|Texas Instruments Incorporated
|IWRL6432 Single-Chip 60GHz mmWave Sensor
[IBIS Ver]   5.0
[Comment Char] |_char
[File name]   iwrl6432_wcsp111.ibs
[Date]   12/10/2024
[File Rev]   1.0
[Source]   Cadence Layout Workbench 22.1.4.12161.401368   004
[Notes]   Revision History:
| Rev 1.0: 12/10/2024
| - Initial version of the model
[Disclaimer]
| This model is designed as an aid for customers of Texas Instruments.
| TI and its licensors and suppliers make no warranties, either expressed
| or implied, with respect to this  model, including the warranties of
| merchantability or fitness for a particular purpose. The model is
| provided solely on an "as is" basis. The entire risk as to its quality
| and performance is with the customer.
| This model is subject to change without notice. Texas Instruments
| Incorporated is not responsible for updating this model.
[Copyright]
(C) Copyright 2024 Texas Instruments Incorporated.All rights reserved.
|  Component IWRL6432BDQGYFFR 111-pin - YFF0111 package
|  Part # IWRL6432BDQGYFFR
[Component]   IWRL6432BDQGYFFR
[Manufacturer]   Texas Instruments
[Package]   |111 WCSP - YFF0111 package
|  variable   typ   min   max
R_pkg   0.12533   0.026709   0.27962
L_pkg   3.002e-10   1.085e-10   5.3e-10
C_pkg   3.033e-13   2.488e-13   4.027e-13
[Pin]   signal_name   model_name   R_pin   L_pin   C_pin
A1   VSSA   GND   NA   NA   NA
A2   TX1   NC   NA   NA   NA
A3   VSSA   GND   NA   NA   NA
A4   TX2   NC   NA   NA   NA
A5   VSSA   GND   NA   NA   NA
A6   VIOIN_18   POWER   NA   NA   NA
A7   VSS   GND   NA   NA   NA
A8   VDD   POWER   NA   NA   NA
A9   QSPI[2]   IO2   NA   NA   NA
A10   QSPI[3]   IO2   NA   NA   NA
A11   VSS   GND   NA   NA   NA
B1   VSSA   GND   NA   NA   NA
B2   VSSA   GND   NA   NA   NA
B4   VSSA   GND   NA   NA   NA
B5   VSSA   GND   NA   NA   NA
B6   VPP   POWER   NA   NA   NA
B7   VSS   GND   NA   NA   NA
B8   VDD   POWER   NA   NA   NA
B9   QSPI_CS   IO2   NA   NA   NA
B10   QSPI[0]   IO2   NA   NA   NA
B11   QSPI[1]   IO2   NA   NA   NA
C1   CLKM   NC   NA   NA   NA
C5   VSSA_PM   NC   NA   NA   NA
C6   VDD   POWER   NA   NA   NA
C7   VDD   POWER   NA   NA   NA
C8   VDD   POWER   NA   NA   NA
C9   SPIA_MOSI   IO2   NA   NA   NA
C10   SPIA_MISO   IO2   NA   NA   NA
C11   QSPI_CLK   IO2   NA   NA   NA
D1   CLKP   NC   NA   NA   NA
D2   VOUT_14SYNTH   NC   NA   NA   NA
D3   VDDA_10RF   POWER   NA   NA   NA
D4   VDDA_10RF   POWER   NA   NA   NA
D5   OSC_CLK_OUT   NC   NA   NA   NA
D6   VDD   POWER   NA   NA   NA
D7   VDD   POWER   NA   NA   NA
D8   VDD   POWER   NA   NA   NA
D9   VDD   POWER   NA   NA   NA
D10   SPIA_CS0_N   IO2   NA   NA   NA
D11   SPIA_CLK   IO2   NA   NA   NA
E1   VSSA   GND   NA   NA   NA
E2   VSSA   GND   NA   NA   NA
E6   VDD   POWER   NA   NA   NA
E7   VDD   POWER   NA   NA   NA
E8   VDD   POWER   NA   NA   NA
E9   VDD   POWER   NA   NA   NA
E10   TCK   IO2   NA   NA   NA
E11   VIOIN   POWER   NA   NA   NA
F1   RX3   NC   NA   NA   NA
F2   VSSA   GND   NA   NA   NA
F3   VDDA_18VCO   POWER   NA   NA   NA
F4   VIN_18PM   POWER   NA   NA   NA
F5   VIOIN_18CLK   POWER   NA   NA   NA
F6   VSS   GND   NA   NA   NA
F7   VSS   GND   NA   NA   NA
F8   VSS   GND   NA   NA   NA
F9   VSS   GND   NA   NA   NA
F10   TDI   IO2   NA   NA   NA
F11   TDO   IO2   NA   NA   NA
G1   VSSA   GND   NA   NA   NA
G2   VSSA   GND   NA   NA   NA
G3   VOUT_14APLL   NC   NA   NA   NA
G4   VDDA_18BB   POWER   NA   NA   NA
G5   VSS   GND   NA   NA   NA
G6   VSS   GND   NA   NA   NA
G7   VSS   GND   NA   NA   NA
G8   VSS   GND   NA   NA   NA
G9   VSS   GND   NA   NA   NA
G10   TMS   IO2   NA   NA   NA
G11   VIOIN_18   POWER   NA   NA   NA
H1   RX2   NC   NA   NA   NA
H2   VSSA   GND   NA   NA   NA
H3   VDDA_10RF   POWER   NA   NA   NA
H4   VBGAP   NC   NA   NA   NA
H6   VSS   GND   NA   NA   NA
H7   VSS   GND   NA   NA   NA
H8   VSS   GND   NA   NA   NA
H9   VSS   GND   NA   NA   NA
H10   RS232_TX   IO2   NA   NA   NA
H11   RS232_RX   IO2   NA   NA   NA
J1   VSSA   GND   NA   NA   NA
J2   VSSA   GND   NA   NA   NA
J3   VDDA_10RF   POWER   NA   NA   NA
J5   GPADC2   NC   NA   NA   NA
J6   VSS   GND   NA   NA   NA
J7   VSS   GND   NA   NA   NA
J8   HOST_CLK_REQ   IO1   NA   NA   NA
J9   GPIO_5   IO1   NA   NA   NA
J10   GPIO_2   IO2   NA   NA   NA
J11   PMIC_CLKOUT   IO2   NA   NA   NA
K1   RX1   NC   NA   NA   NA
K2   VSSA   GND   NA   NA   NA
K3   VDDA_12RF   POWER   NA   NA   NA
K5   GPADC1   NC   NA   NA   NA
K6   VDD   POWER   NA   NA   NA
K7   VIOIN_18   POWER   NA   NA   NA
K8   NRESET   IOOD   NA   NA   NA
K9   UARTA_RTS   IO1   NA   NA   NA
K10   NERROR_OUT   IO1   NA   NA   NA
K11   UARTA_RX   IO1   NA   NA   NA
L1   VSSA   GND   NA   NA   NA
L2   VSSA   GND   NA   NA   NA
L3   VDDA_12RF   POWER   NA   NA   NA
L4   VDDA_18BB   POWER   NA   NA   NA
L5   VDDA_18BB   POWER   NA   NA   NA
L6   VDD_SRAM   POWER   NA   NA   NA
L7   VIOIN_18   POWER   NA   NA   NA
L8   VNWA   POWER   NA   NA   NA
L9   VIOIN   POWER   NA   NA   NA
L10   UARTA_TX   IO1   NA   NA   NA
L11   VSS   GND   NA   NA   NA
| Model IOOD
[Model Selector] IOOD
|SC1 IS A SLEW RATE CONTROL PIN
|5% SUPPLY VARIATION MODES WITH 1.8V NOM SUPPLY
IOOD_V_PUPDOFF_5P_SC1_1P8  Cell operated at 1.8(nom)
|IOOD_V_PUPDOFF_5P_SC1_1P8; BUFFER WITH WEAK PULUP/PULLDOWN OFF AT 5% SUPPLY
|VARIATION WITH SC1=1 MEANING SLOW MODE OF OPERATION
IOOD_V_PD_ON_5P_!SC1_1P8  Cell operated at 1.8(nom)
|IOOD_V_PD_ON_5P_!SC1_1P8; BUFFER WITH WEAK_PULLDOWN_ON AT 5% SUPPLY
|VARIATION WITH SC1=0 MEANING FAST MODE OF OPERATION
IOOD_V_PD_ON_5P_SC1_1P8  Cell operated at 1.8(nom)
|IOOD_V_PD_ON_5P_SC1_1P8; BUFFER WITH WEAK_PULLDOWN_ON AT 5% SUPPLY
|VARIATION WITH SC1=1 MEANING SLOW MODE OF OPERATION
IOOD_V_PU_ON_5P_!SC1_1P8  Cell operated at 1.8(nom)
|IOOD_V_PU_ON_5P_!SC1_1P8; BUFFER WITH WEAK_PULLUP_ON AT 5% SUPPLY
|VARIATION WITH SC1=0 MEANING FAST MODE OF OPERATION
IOOD_V_PUPDOFF_5P_!SC1_1P8  Cell operated at 1.8(nom)
|IOOD_V_PUPDOFF_5P_!SC1_1P8; BUFFER WITH WEAK PULUP/PULLDOWN OFF AT 5% SUPPLY
|VARIATION WITH SC1=0 MEANING FAST MODE OF OPERATION
IOOD_V_PU_ON_5P_SC1_1P8  Cell operated at 1.8(nom)
|IOOD_V_PU_ON_5P_SC1_1P8; BUFFER WITH WEAK_PULLUP_ON AT 5% SUPPLY
|VARIATION WITH SC1=1 MEANING SLOW MODE OF OPERATION
|5% SUPPLY VARIATION MODES WITH 3.3V NOM SUPPLY
IOOD_V_PUPDOFF_5P_SC1_3P3  Cell operated at 3.3(nom)
|IOOD_V_PUPDOFF_5P_SC1_3P3; BUFFER WITH WEAK PULUP/PULLDOWN OFF AT 5% SUPPLY
|VARIATION WITH SC1=1 MEANING SLOW MODE OF OPERATION
IOOD_V_PD_ON_5P_!SC1_3P3  Cell operated at 3.3(nom)
|IOOD_V_PD_ON_5P_!SC1_3P3; BUFFER WITH WEAK_PULLDOWN_ON AT 5% SUPPLY
|VARIATION WITH SC1=0 MEANING FAST MODE OF OPERATION
IOOD_V_PD_ON_5P_SC1_3P3  Cell operated at 3.3(nom)
|IOOD_V_PD_ON_5P_SC1_3P3; BUFFER WITH WEAK_PULLDOWN_ON AT 5% SUPPLY
|VARIATION WITH SC1=1 MEANING SLOW MODE OF OPERATION
IOOD_V_PU_ON_5P_!SC1_3P3  Cell operated at 3.3(nom)
|IOOD_V_PU_ON_5P_!SC1_3P3; BUFFER WITH WEAK_PULLUP_ON AT 5% SUPPLY
|VARIATION WITH SC1=0 MEANING FAST MODE OF OPERATION
IOOD_V_PUPDOFF_5P_!SC1_3P3  Cell operated at 3.3(nom)
|IOOD_V_PUPDOFF_5P_!SC1_3P3; BUFFER WITH WEAK PULUP/PULLDOWN OFF AT 5% SUPPLY
|VARIATION WITH SC1=0 MEANING FAST MODE OF OPERATION
IOOD_V_PU_ON_5P_SC1_3P3  Cell operated at 3.3(nom)
|IOOD_V_PU_ON_5P_SC1_3P3; BUFFER WITH WEAK_PULLUP_ON AT 5% SUPPLY
|VARIATION WITH SC1=1 MEANING SLOW MODE OF OPERATION
| 10% SUPPLY VARIATION MODES WITH 1.8V NOM SUPPLY
IOOD_V_PUPDOFF_10P_SC1_1P8  Cell operated at 1.8(nom)
|IOOD_V_PUPDOFF_10P_SC1_1P8; BUFFER WITH WEAK PULUP/PULLDOWN OFF AT 10% SUPPLY
|VARIATION WITH SC1=1 MEANING SLOW MODE OF OPERATION
IOOD_V_PD_ON_10P_!SC1_1P8  Cell operated at 1.8(nom)
|IOOD_V_PD_ON_10P_!SC1_1P8; BUFFER WITH WEAK_PULLDOWN_ON AT 10% SUPPLY
|VARIATION WITH SC1=0 MEANING FAST MODE OF OPERATION
IOOD_V_PD_ON_10P_SC1_1P8  Cell operated at 1.8(nom)
|IOOD_V_PD_ON_10P_SC1_1P8; BUFFER WITH WEAK_PULLDOWN_ON AT 10% SUPPLY
|VARIATION WITH SC1=1 MEANING SLOW MODE OF OPERATION
IOOD_V_PU_ON_10P_!SC1_1P8  Cell operated at 1.8(nom)
|IOOD_V_PU_ON_10P_!SC1_1P8; BUFFER WITH WEAK_PULLUP_ON AT 10% SUPPLY
|VARIATION WITH SC1=0 MEANING FAST MODE OF OPERATION
IOOD_V_PUPDOFF_10P_!SC1_1P8  Cell operated at 1.8(nom)
|IOOD_V_PUPDOFF_10P_!SC1_1P8; BUFFER WITH WEAK PULUP/PULLDOWN OFF AT 10% SUPPLY
|VARIATION WITH SC1=0 MEANING FAST MODE OF OPERATION
IOOD_V_PU_ON_10P_SC1_1P8  Cell operated at 1.8(nom)
|IOOD_V_PU_ON_10P_SC1_1P8; BUFFER WITH WEAK_PULLUP_ON AT 10% SUPPLY
|VARIATION WITH SC1=1 MEANING SLOW MODE OF OPERATION
| 10% SUPPLY VARIATION MODES WITH 3.3V NOM SUPPLY
IOOD_V_PUPDOFF_10P_SC1_3P3  Cell operated at 3.3(nom)
|IOOD_V_PUPDOFF_10P_SC1_3P3; BUFFER WITH WEAK PULUP/PULLDOWN OFF AT 10% SUPPLY
|VARIATION WITH SC1=1 MEANING SLOW MODE OF OPERATION
IOOD_V_PD_ON_10P_!SC1_3P3  Cell operated at 3.3(nom)
|IOOD_V_PD_ON_10P_!SC1_3P3; BUFFER WITH WEAK_PULLDOWN_ON 10% SUPPLY
|VARIATION WITH SC1=0 MEANING FAST MODE OF OPERATION
IOOD_V_PD_ON_10P_SC1_3P3  Cell operated at 3.3(nom)
|IOOD_V_PD_ON_10P_SC1_3P3; BUFFER WITH WEAK_PULLDOWN_ON AT 10% SUPPLY
|VARIATION WITH SC1=1 MEANING SLOW MODE OF OPERATION
IOOD_V_PU_ON_10P_!SC1_3P3  Cell operated at 3.3(nom)
|IOOD_V_PU_ON_10P_!SC1_3P3; BUFFER WITH WEAK_PULLUP_ON AT 10% SUPPLY
|VARIATION WITH SC1=0 MEANING FAST MODE OF OPERATION
IOOD_V_PUPDOFF_10P_!SC1_3P3  Cell operated at 3.3(nom)
|IOOD_V_PUPDOFF_10P_!SC1_3P3; BUFFER WITH WEAK PULUP/PULLDOWN OFF AT 10% SUPPLY
|VARIATION WITH SC1=0 MEANING FAST MODE OF OPERATION
IOOD_V_PU_ON_10P_SC1_3P3  Cell operated at 3.3(nom)
|IOOD_V_PU_ON_10P_SC1_3P3; BUFFER WITH WEAK_PULLUP_ON AT 10% SUPPLY
|VARIATION WITH SC1=1 MEANING SLOW MODE OF OPERATION
| Model IO1
[Model Selector] IO1
|SC1 IS A SLEW RATE CONTROL PIN
|5% SUPPLY VARIATION MODES WITH 1.8V NOM SUPPLY
BC40D_V_PUPDOFF_5P_SC1_1P8  Cell operated at 1.8(nom)
|BC40D_V_PUPDOFF_5P_SC1_1P8; BUFFER WITH WEAK PULUP/PULLDOWN OFF AT 5% SUPPLY
|VARIATION WITH SC1=1 MEANING SLOW MODE OF OPERATION
BC40D_V_PD_ON_5P_!SC1_1P8  Cell operated at 1.8(nom)
|BC40D_V_PD_ON_5P_!SC1_1P8; BUFFER WITH WEAK_PULLDOWN_ON AT 5% SUPPLY
|VARIATION WITH SC1=0 MEANING FAST MODE OF OPERATION
BC40D_V_PD_ON_5P_SC1_1P8  Cell operated at 1.8(nom)
|BC40D_V_PD_ON_5P_SC1_1P8; BUFFER WITH WEAK_PULLDOWN_ON AT 5% SUPPLY
|VARIATION WITH SC1=1 MEANING SLOW MODE OF OPERATION
BC40D_V_PU_ON_5P_!SC1_1P8  Cell operated at 1.8(nom)
|BC40D_V_PU_ON_5P_!SC1_1P8; BUFFER WITH WEAK_PULLUP_ON AT 5% SUPPLY
|VARIATION WITH SC1=0 MEANING FAST MODE OF OPERATION
BC40D_V_PUPDOFF_5P_!SC1_1P8  Cell operated at 1.8(nom)
|BC40D_V_PUPDOFF_5P_!SC1_1P8; BUFFER WITH WEAK PULUP/PULLDOWN OFF AT 5% SUPPLY
|VARIATION WITH SC1=0 MEANING FAST MODE OF OPERATION
BC40D_V_PU_ON_5P_SC1_1P8  Cell operated at 1.8(nom)
|BC40D_V_PU_ON_5P_SC1_1P8; BUFFER WITH WEAK_PULLUP_ON AT 5% SUPPLY
|VARIATION WITH SC1=1 MEANING SLOW MODE OF OPERATION
|5% SUPPLY VARIATION MODES WITH 3.3V NOM SUPPLY
BC40D_V_PUPDOFF_5P_SC1_3P3  Cell operated at 3.3(nom)
|BC40D_V_PUPDOFF_5P_SC1_3P3; BUFFER WITH WEAK PULUP/PULLDOWN OFF AT 5% SUPPLY
|VARIATION WITH SC1=1 MEANING SLOW MODE OF OPERATION
BC40D_V_PD_ON_5P_!SC1_3P3  Cell operated at 3.3(nom)
|BC40D_V_PD_ON_5P_!SC1_3P3; BUFFER WITH WEAK_PULLDOWN_ON AT 5% SUPPLY
|VARIATION WITH SC1=0 MEANING FAST MODE OF OPERATION
BC40D_V_PD_ON_5P_SC1_3P3  Cell operated at 3.3(nom)
|BC40D_V_PD_ON_5P_SC1_3P3; BUFFER WITH WEAK_PULLDOWN_ON AT 5% SUPPLY
|VARIATION WITH SC1=1 MEANING SLOW MODE OF OPERATION
BC40D_V_PU_ON_5P_!SC1_3P3  Cell operated at 3.3(nom)
|BC40D_V_PU_ON_5P_!SC1_3P3; BUFFER WITH WEAK_PULLUP_ON AT 5% SUPPLY
|VARIATION WITH SC1=0 MEANING FAST MODE OF OPERATION
BC40D_V_PUPDOFF_5P_!SC1_3P3  Cell operated at 3.3(nom)
|BC40D_V_PUPDOFF_5P_!SC1_3P3; BUFFER WITH WEAK PULUP/PULLDOWN OFF AT 5% SUPPLY
|VARIATION WITH SC1=0 MEANING FAST MODE OF OPERATION
BC40D_V_PU_ON_5P_SC1_3P3  Cell operated at 3.3(nom)
|BC40D_V_PU_ON_5P_SC1_3P3; BUFFER WITH WEAK_PULLUP_ON AT 5% SUPPLY
|VARIATION WITH SC1=1 MEANING SLOW MODE OF OPERATION
| 10% SUPPLY VARIATION MODES WITH 1.8V NOM SUPPLY
BC40D_V_PUPDOFF_10P_SC1_1P8  Cell operated at 1.8(nom)
|BC40D_V_PUPDOFF_10P_SC1_1P8; BUFFER WITH WEAK PULUP/PULLDOWN OFF AT 10% SUPPLY
|VARIATION WITH SC1=1 MEANING SLOW MODE OF OPERATION
BC40D_V_PD_ON_10P_!SC1_1P8  Cell operated at 1.8(nom)
|BC40D_V_PD_ON_10P_!SC1_1P8; BUFFER WITH WEAK_PULLDOWN_ON AT 10% SUPPLY
|VARIATION WITH SC1=0 MEANING FAST MODE OF OPERATION
BC40D_V_PD_ON_10P_SC1_1P8  Cell operated at 1.8(nom)
|BC40D_V_PD_ON_10P_SC1_1P8; BUFFER WITH WEAK_PULLDOWN_ON AT 10% SUPPLY
|VARIATION WITH SC1=1 MEANING SLOW MODE OF OPERATION
BC40D_V_PU_ON_10P_!SC1_1P8  Cell operated at 1.8(nom)
|BC40D_V_PU_ON_10P_!SC1_1P8; BUFFER WITH WEAK_PULLUP_ON AT 10% SUPPLY
|VARIATION WITH SC1=0 MEANING FAST MODE OF OPERATION
BC40D_V_PUPDOFF_10P_!SC1_1P8  Cell operated at 1.8(nom)
|BC40D_V_PUPDOFF_10P_!SC1_1P8; BUFFER WITH WEAK PULUP/PULLDOWN OFF AT 10% SUPPLY
|VARIATION WITH SC1=0 MEANING FAST MODE OF OPERATION
BC40D_V_PU_ON_10P_SC1_1P8  Cell operated at 1.8(nom)
|BC40D_V_PU_ON_10P_SC1_1P8; BUFFER WITH WEAK_PULLUP_ON AT 10% SUPPLY
|VARIATION WITH SC1=1 MEANING SLOW MODE OF OPERATION
| 10% SUPPLY VARIATION MODES WITH 3.3V NOM SUPPLY
BC40D_V_PUPDOFF_10P_SC1_3P3  Cell operated at 3.3(nom)
|BC40D_V_PUPDOFF_10P_SC1_3P3; BUFFER WITH WEAK PULUP/PULLDOWN OFF AT 10% SUPPLY
|VARIATION WITH SC1=1 MEANING SLOW MODE OF OPERATION
BC40D_V_PD_ON_10P_!SC1_3P3  Cell operated at 3.3(nom)
|BC40D_V_PD_ON_10P_!SC1_3P3; BUFFER WITH WEAK_PULLDOWN_ON 10% SUPPLY
|VARIATION WITH SC1=0 MEANING FAST MODE OF OPERATION
BC40D_V_PD_ON_10P_SC1_3P3  Cell operated at 3.3(nom)
|BC40D_V_PD_ON_10P_SC1_3P3; BUFFER WITH WEAK_PULLDOWN_ON AT 10% SUPPLY
|VARIATION WITH SC1=1 MEANING SLOW MODE OF OPERATION
BC40D_V_PU_ON_10P_!SC1_3P3  Cell operated at 3.3(nom)
|BC40D_V_PU_ON_10P_!SC1_3P3; BUFFER WITH WEAK_PULLUP_ON AT 10% SUPPLY
|VARIATION WITH SC1=0 MEANING FAST MODE OF OPERATION
BC40D_V_PUPDOFF_10P_!SC1_3P3  Cell operated at 3.3(nom)
|BC40D_V_PUPDOFF_10P_!SC1_3P3; BUFFER WITH WEAK PULUP/PULLDOWN OFF AT 10% SUPPLY
|VARIATION WITH SC1=0 MEANING FAST MODE OF OPERATION
BC40D_V_PU_ON_10P_SC1_3P3  Cell operated at 3.3(nom)
|BC40D_V_PU_ON_10P_SC1_3P3; BUFFER WITH WEAK_PULLUP_ON AT 10% SUPPLY
|VARIATION WITH SC1=1 MEANING SLOW MODE OF OPERATION
| Model IO2
[Model Selector] IO2
|SC1 IS A SLEW RATE CONTROL PIN
|5% SUPPLY VARIATION MODES WITH 1.8V NOM SUPPLY
BC40D_H_PUPDOFF_5P_SC1_1P8  Cell operated at 1.8(nom)
|BC40D_H_PUPDOFF_5P_SC1_1P8; BUFFER WITH WEAK PULUP/PULLDOWN OFF AT 5% SUPPLY
|VARIATION WITH SC1=1 MEANING SLOW MODE OF OPERATION
BC40D_H_PD_ON_5P_!SC1_1P8  Cell operated at 1.8(nom)
|BC40D_H_PD_ON_5P_!SC1_1P8; BUFFER WITH WEAK_PULLDOWN_ON AT 5% SUPPLY
|VARIATION WITH SC1=0 MEANING FAST MODE OF OPERATION
BC40D_H_PD_ON_5P_SC1_1P8  Cell operated at 1.8(nom)
|BC40D_H_PD_ON_5P_SC1_1P8; BUFFER WITH WEAK_PULLDOWN_ON AT 5% SUPPLY
|VARIATION WITH SC1=1 MEANING SLOW MODE OF OPERATION
BC40D_H_PU_ON_5P_!SC1_1P8  Cell operated at 1.8(nom)
|BC40D_H_PU_ON_5P_!SC1_1P8; BUFFER WITH WEAK_PULLUP_ON AT 5% SUPPLY
|VARIATION WITH SC1=0 MEANING FAST MODE OF OPERATION
BC40D_H_PUPDOFF_5P_!SC1_1P8  Cell operated at 1.8(nom)
|BC40D_H_PUPDOFF_5P_!SC1_1P8; BUFFER WITH WEAK PULUP/PULLDOWN OFF AT 5% SUPPLY
|VARIATION WITH SC1=0 MEANING FAST MODE OF OPERATION
BC40D_H_PU_ON_5P_SC1_1P8  Cell operated at 1.8(nom)
|BC40D_H_PU_ON_5P_SC1_1P8; BUFFER WITH WEAK_PULLUP_ON AT 5% SUPPLY
|VARIATION WITH SC1=1 MEANING SLOW MODE OF OPERATION
|5% SUPPLY VARIATION MODES WITH 3.3V NOM SUPPLY
BC40D_H_PUPDOFF_5P_SC1_3P3  Cell operated at 3.3(nom)
|BC40D_H_PUPDOFF_5P_SC1_3P3; BUFFER WITH WEAK PULUP/PULLDOWN OFF AT 5% SUPPLY
|VARIATION WITH SC1=1 MEANING SLOW MODE OF OPERATION
BC40D_H_PD_ON_5P_!SC1_3P3  Cell operated at 3.3(nom)
|BC40D_H_PD_ON_5P_!SC1_3P3; BUFFER WITH WEAK_PULLDOWN_ON AT 5% SUPPLY
|VARIATION WITH SC1=0 MEANING FAST MODE OF OPERATION
BC40D_H_PD_ON_5P_SC1_3P3  Cell operated at 3.3(nom)
|BC40D_H_PD_ON_5P_SC1_3P3; BUFFER WITH WEAK_PULLDOWN_ON AT 5% SUPPLY
|VARIATION WITH SC1=1 MEANING SLOW MODE OF OPERATION
BC40D_H_PU_ON_5P_!SC1_3P3  Cell operated at 3.3(nom)
|BC40D_H_PU_ON_5P_!SC1_3P3; BUFFER WITH WEAK_PULLUP_ON AT 5% SUPPLY
|VARIATION WITH SC1=0 MEANING FAST MODE OF OPERATION
BC40D_H_PUPDOFF_5P_!SC1_3P3  Cell operated at 3.3(nom)
|BC40D_H_PUPDOFF_5P_!SC1_3P3; BUFFER WITH WEAK PULUP/PULLDOWN OFF AT 5% SUPPLY
|VARIATION WITH SC1=0 MEANING FAST MODE OF OPERATION
BC40D_H_PU_ON_5P_SC1_3P3  Cell operated at 3.3(nom)
|BC40D_H_PU_ON_5P_SC1_3P3; BUFFER WITH WEAK_PULLUP_ON AT 5% SUPPLY
|VARIATION WITH SC1=1 MEANING SLOW MODE OF OPERATION
| 10% SUPPLY VARIATION MODES WITH 1.8V NOM SUPPLY
BC40D_H_PUPDOFF_10P_SC1_1P8  Cell operated at 1.8(nom)
|BC40D_H_PUPDOFF_10P_SC1_1P8; BUFFER WITH WEAK PULUP/PULLDOWN OFF AT 10% SUPPLY
|VARIATION WITH SC1=1 MEANING SLOW MODE OF OPERATION
BC40D_H_PD_ON_10P_!SC1_1P8  Cell operated at 1.8(nom)
|BC40D_H_PD_ON_10P_!SC1_1P8; BUFFER WITH WEAK_PULLDOWN_ON AT 10% SUPPLY
|VARIATION WITH SC1=0 MEANING FAST MODE OF OPERATION
BC40D_H_PD_ON_10P_SC1_1P8  Cell operated at 1.8(nom)
|BC40D_H_PD_ON_10P_SC1_1P8; BUFFER WITH WEAK_PULLDOWN_ON AT 10% SUPPLY
|VARIATION WITH SC1=1 MEANING SLOW MODE OF OPERATION
BC40D_H_PU_ON_10P_!SC1_1P8  Cell operated at 1.8(nom)
|BC40D_H_PU_ON_10P_!SC1_1P8; BUFFER WITH WEAK_PULLUP_ON AT 10% SUPPLY
|VARIATION WITH SC1=0 MEANING FAST MODE OF OPERATION
BC40D_H_PUPDOFF_10P_!SC1_1P8  Cell operated at 1.8(nom)
|BC40D_H_PUPDOFF_10P_!SC1_1P8; BUFFER WITH WEAK PULUP/PULLDOWN OFF AT 10% SUPPLY
|VARIATION WITH SC1=0 MEANING FAST MODE OF OPERATION
BC40D_H_PU_ON_10P_SC1_1P8  Cell operated at 1.8(nom)
|BC40D_H_PU_ON_10P_SC1_1P8; BUFFER WITH WEAK_PULLUP_ON AT 10% SUPPLY
|VARIATION WITH SC1=1 MEANING SLOW MODE OF OPERATION
| 10% SUPPLY VARIATION MODES WITH 3.3V NOM SUPPLY
BC40D_H_PUPDOFF_10P_SC1_3P3  Cell operated at 3.3(nom)
|BC40D_H_PUPDOFF_10P_SC1_3P3; BUFFER WITH WEAK PULUP/PULLDOWN OFF AT 10% SUPPLY
|VARIATION WITH SC1=1 MEANING SLOW MODE OF OPERATION
BC40D_H_PD_ON_10P_!SC1_3P3  Cell operated at 3.3(nom)
|BC40D_H_PD_ON_10P_!SC1_3P3; BUFFER WITH WEAK_PULLDOWN_ON 10% SUPPLY
|VARIATION WITH SC1=0 MEANING FAST MODE OF OPERATION
BC40D_H_PD_ON_10P_SC1_3P3  Cell operated at 3.3(nom)
|BC40D_H_PD_ON_10P_SC1_3P3; BUFFER WITH WEAK_PULLDOWN_ON AT 10% SUPPLY
|VARIATION WITH SC1=1 MEANING SLOW MODE OF OPERATION
BC40D_H_PU_ON_10P_!SC1_3P3  Cell operated at 3.3(nom)
|BC40D_H_PU_ON_10P_!SC1_3P3; BUFFER WITH WEAK_PULLUP_ON AT 10% SUPPLY
|VARIATION WITH SC1=0 MEANING FAST MODE OF OPERATION
BC40D_H_PUPDOFF_10P_!SC1_3P3  Cell operated at 3.3(nom)
|BC40D_H_PUPDOFF_10P_!SC1_3P3; BUFFER WITH WEAK PULUP/PULLDOWN OFF AT 10% SUPPLY
|VARIATION WITH SC1=0 MEANING FAST MODE OF OPERATION
BC40D_H_PU_ON_10P_SC1_3P3  Cell operated at 3.3(nom)
[Define Package Model]   IWRL6432BDQGYFFR
[Manufacturer]   TI
[OEM]   TI
[Description]   WCSP
|[Number of Sections]   1
[Number of Pins]   32
[Pin Numbers]
|[Pin Name]  Net Number   Net Name   Net's All Pins
K6   | 1   VDD   K6
   |A8
   |E7
   |E6
   |D6
   |C6
   |C7
   |D7
   |E8
   |C8
   |D8
   |B8
   |E9
   |D9
L6   | 2   VDD_SRAM   L6
E11   | 3   VIOIN   E11
   |L9
A6   | 4   VIOIN_18   A6
   |K7
   |L7
   |G11
L8   | 5   VNWA   L8
B6   | 6   VPP   B6
J10   | 7   GPIO_2   J10
J9   | 8   GPIO_5   J9
J8   | 9   HOST_CLK_REQ   J8
K10   | 10   NERROR_OUT   K10
K8   | 11   NRESET   K8
D5   | 12   OSC_CLK_OUT   D5
J11   | 13   PMIC_CLKOUT   J11
B10   | 14   QSPI[0]   B10
B11   | 15   QSPI[1]   B11
A9   | 16   QSPI[2]   A9
A10   | 17   QSPI[3]   A10
C11   | 18   QSPI_CLK   C11
B9   | 19   QSPI_CS   B9
H11   | 20   RS232_RX   H11
H10   | 21   RS232_TX   H10
D11   | 22   SPIA_CLK   D11
D10   | 23   SPIA_CS0_N   D10
C10   | 24   SPIA_MISO   C10
C9   | 25   SPIA_MOSI   C9
E10   | 26   TCK   E10
F10   | 27   TDI   F10
F11   | 28   TDO   F11
G10   | 29   TMS   G10
K9   | 30   UARTA_RTS   K9
K11   | 31   UARTA_RX   K11
L10   | 32   UARTA_TX   L10
[Model Data]
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[End Model Data]
[End Package Model]
| Models and submodels in the file (72): BC40D_V_PUPDOFF_5P_SC1_1P8 (I/O), BC40D_V_PD_ON_5P_!SC1_1P8 (I/O), BC40D_V_PD_ON_5P_SC1_1P8 (I/O), BC40D_V_PU_ON_5P_!SC1_1P8 (I/O), BC40D_V_PUPDOFF_5P_!SC1_1P8 (I/O), BC40D_V_PU_ON_5P_SC1_1P8 (I/O), BC40D_V_PUPDOFF_5P_SC1_3P3 (I/O), BC40D_V_PD_ON_5P_!SC1_3P3 (I/O), BC40D_V_PD_ON_5P_SC1_3P3 (I/O), BC40D_V_PU_ON_5P_!SC1_3P3 (I/O), BC40D_V_PUPDOFF_5P_!SC1_3P3 (I/O), BC40D_V_PU_ON_5P_SC1_3P3 (I/O), BC40D_V_PUPDOFF_10P_SC1_1P8 (I/O), BC40D_V_PD_ON_10P_!SC1_1P8 (I/O), BC40D_V_PD_ON_10P_SC1_1P8 (I/O), BC40D_V_PU_ON_10P_!SC1_1P8 (I/O), BC40D_V_PUPDOFF_10P_!SC1_1P8 (I/O), BC40D_V_PU_ON_10P_SC1_1P8 (I/O), BC40D_V_PUPDOFF_10P_SC1_3P3 (I/O), BC40D_V_PD_ON_10P_!SC1_3P3 (I/O), BC40D_V_PD_ON_10P_SC1_3P3 (I/O), BC40D_V_PU_ON_10P_!SC1_3P3 (I/O), BC40D_V_PUPDOFF_10P_!SC1_3P3 (I/O), BC40D_V_PU_ON_10P_SC1_3P3 (I/O), BC40D_H_PUPDOFF_5P_SC1_1P8 (I/O), BC40D_H_PD_ON_5P_!SC1_1P8 (I/O), BC40D_H_PD_ON_5P_SC1_1P8 (I/O), BC40D_H_PU_ON_5P_!SC1_1P8 (I/O), BC40D_H_PUPDOFF_5P_!SC1_1P8 (I/O), BC40D_H_PU_ON_5P_SC1_1P8 (I/O), BC40D_H_PUPDOFF_5P_SC1_3P3 (I/O), BC40D_H_PD_ON_5P_!SC1_3P3 (I/O), BC40D_H_PD_ON_5P_SC1_3P3 (I/O), BC40D_H_PU_ON_5P_!SC1_3P3 (I/O), BC40D_H_PUPDOFF_5P_!SC1_3P3 (I/O), BC40D_H_PU_ON_5P_SC1_3P3 (I/O), BC40D_H_PUPDOFF_10P_SC1_1P8 (I/O), BC40D_H_PD_ON_10P_!SC1_1P8 (I/O), BC40D_H_PD_ON_10P_SC1_1P8 (I/O), BC40D_H_PU_ON_10P_!SC1_1P8 (I/O), BC40D_H_PUPDOFF_10P_!SC1_1P8 (I/O), BC40D_H_PU_ON_10P_SC1_1P8 (I/O), BC40D_H_PUPDOFF_10P_SC1_3P3 (I/O), BC40D_H_PD_ON_10P_!SC1_3P3 (I/O), BC40D_H_PD_ON_10P_SC1_3P3 (I/O), BC40D_H_PU_ON_10P_!SC1_3P3 (I/O), BC40D_H_PUPDOFF_10P_!SC1_3P3 (I/O), BC40D_H_PU_ON_10P_SC1_3P3 (I/O), IOOD_V_PUPDOFF_5P_SC1_1P8 (I/O_open_drain), IOOD_V_PD_ON_5P_!SC1_1P8 (I/O_open_drain), IOOD_V_PD_ON_5P_SC1_1P8 (I/O_open_drain), IOOD_V_PU_ON_5P_!SC1_1P8 (I/O_open_drain), IOOD_V_PUPDOFF_5P_!SC1_1P8 (I/O_open_drain), IOOD_V_PU_ON_5P_SC1_1P8 (I/O_open_drain), IOOD_V_PUPDOFF_5P_SC1_3P3 (I/O_open_drain), IOOD_V_PD_ON_5P_!SC1_3P3 (I/O_open_drain), IOOD_V_PD_ON_5P_SC1_3P3 (I/O_open_drain), IOOD_V_PU_ON_5P_!SC1_3P3 (I/O_open_drain), IOOD_V_PUPDOFF_5P_!SC1_3P3 (I/O_open_drain), IOOD_V_PU_ON_5P_SC1_3P3 (I/O_open_drain), IOOD_V_PUPDOFF_10P_SC1_1P8 (I/O_open_drain), IOOD_V_PD_ON_10P_!SC1_1P8 (I/O_open_drain), IOOD_V_PD_ON_10P_SC1_1P8 (I/O_open_drain), IOOD_V_PU_ON_10P_!SC1_1P8 (I/O_open_drain), IOOD_V_PUPDOFF_10P_!SC1_1P8 (I/O_open_drain), IOOD_V_PU_ON_10P_SC1_1P8 (I/O_open_drain), IOOD_V_PUPDOFF_10P_SC1_3P3 (I/O_open_drain), IOOD_V_PD_ON_10P_!SC1_3P3 (I/O_open_drain), IOOD_V_PD_ON_10P_SC1_3P3 (I/O_open_drain), IOOD_V_PU_ON_10P_!SC1_3P3 (I/O_open_drain), IOOD_V_PUPDOFF_10P_!SC1_3P3 (I/O_open_drain), IOOD_V_PU_ON_10P_SC1_3P3 (I/O_open_drain)
